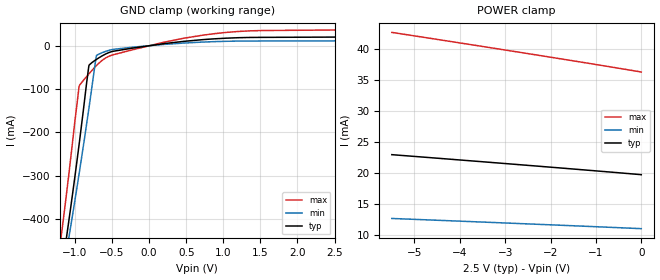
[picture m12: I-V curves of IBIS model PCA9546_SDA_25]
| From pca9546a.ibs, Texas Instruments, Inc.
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[Model]   PCA9546_SDA_25
Model_type  Terminator
| variable   typ   min   max
C_comp   6.36pF   4.76pF   8.41pF
| C_tri-state   6.36pF   4.76pF   8.41pF
[Temperature Range]   40   100   -40
| Ambient temperature   25   85   -40
[Voltage range]   2.5   2.3   2.7
[GND Clamp]
| PCA9546_SDA_25
|   Voltage   I(typ)   I(min)   I(max)
-5.5V     -4.129A    -3.957A    -4.325A
-1.205V   -546.7mA   -566mA     -464.7mA
-1.165V   -501mA     -526.3mA   -411.4mA
-1.105V   -430.4mA   -465.6mA   -328.2mA
-1.08V    -400.3mA   -439.9mA   -292.2mA
-1.055V   -369.7mA   -413.9mA   -255.5mA
-945mV    -228.4mA   -295.9mA   -94.39mA
-810mV    -44.84mA   -141.7mA   -64.62mA
-710mV    -31.63mA   -22.68mA   -45.67mA
-490mV    -13.06mA   -8.634mA   -21.19mA
720mV     13.82mA    8.232mA    24.07mA
2.5V      19.72mA    11.06mA    36.08mA
[POWER Clamp]
| PCA9546_SDA_25
|   Voltage   I(typ)   I(min)   I(max)
-5.5V     22.96mA    12.64mA    42.73mA
-2.385V   21.16mA    11.73mA    39.17mA
-1.055V   20.37mA    11.33mA    37.6mA
-95.1fV   19.72mA    10.99mA    36.33mA
